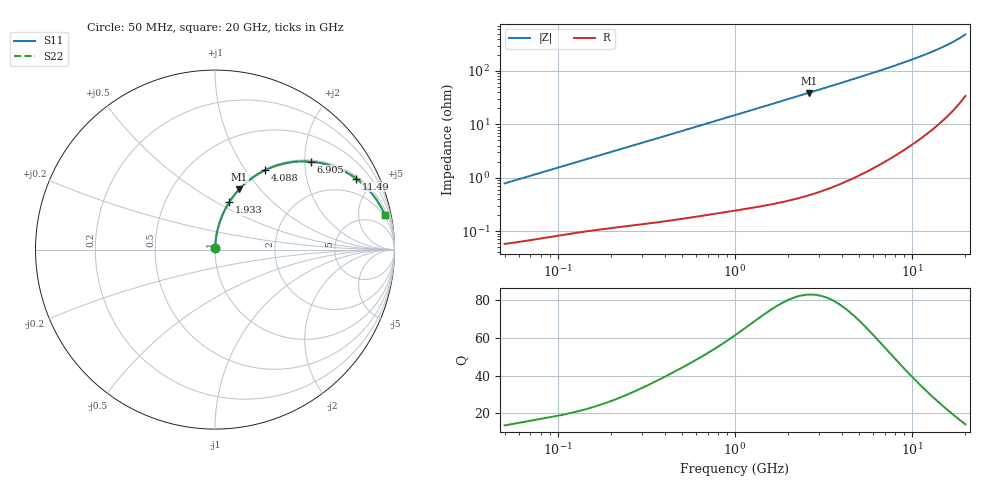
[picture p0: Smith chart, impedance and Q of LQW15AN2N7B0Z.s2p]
!Murata Part Number: LQW15AN2N7B0Z
!These Parameters are Measured in Series Mode Connection
!  o--[Z]--o
!Port1  Port2
!  o-------o
!Freq. Start=50[MHz] Stop=20[GHz], 401[Steps]
# Hz S RI R 50
!Freq.(Hz) S11(Real) S11(Imag) S21(Real) S21(Imag) S12(Real) S12(Imag) S22(Real) S22(Imag)
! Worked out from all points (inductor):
!   401 points, 50 MHz to 20 GHz, reference 50 ohm
!   read as one part in series: L = 2.48 nH near 51.52 MHz
!   highest Q = 83 at 2.608 GHz (marker M1), where L = 2.38 nH
!   S11 on the Smith chart (normalised r, x): 50 MHz: 1.00, +0.02; 1.933 GHz: 1.01, +0.58; 4.088 GHz: 1.02, +1.23; 6.905 GHz: 1.04, +2.15; 11.49 GHz: 1.12, +3.91; 20 GHz: 1.68, +9.64
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5e7  0.000638 0.00782  0.9994 -0.00782  0.9994 -0.00782  0.000638 0.00782
1.364002e8  0.0014 0.0208  0.9986 -0.0208  0.9986 -0.0208  0.0014 0.0208
2.33884e8  0.00246 0.0353  0.9975 -0.0353  0.9975 -0.0353  0.00246 0.0353
3.721004e8  0.00459 0.0556  0.9954 -0.0556  0.9954 -0.0556  0.00459 0.0556
6.285508e8  0.0106 0.0929  0.9894 -0.0929  0.9894 -0.0929  0.0106 0.0929
1e9  0.024 0.1453  0.976 -0.1453  0.976 -0.1453  0.024 0.1453
1.432596e9  0.0462 0.2031  0.9538 -0.2031  0.9538 -0.2031  0.0462 0.2031
1.932977e9  0.0795 0.2644  0.9205 -0.2644  0.9205 -0.2644  0.0795 0.2644
2.608132e9  0.1349 0.3356  0.8651 -0.3356  0.8651 -0.3356  0.1349 0.3356
2.728004e9  0.1457 0.3468  0.8543 -0.3468  0.8543 -0.3468  0.1457 0.3468
3.364474e9  0.2061 0.3984  0.7939 -0.3984  0.7939 -0.3984  0.2061 0.3984
4.087748e9  0.278 0.4415  0.722 -0.4415  0.722 -0.4415  0.278 0.4415
5.433528e9  0.4092 0.4842  0.5908 -0.4842  0.5908 -0.4842  0.4092 0.4842
6.905011e9  0.535 0.4899  0.465 -0.4899  0.465 -0.4899  0.535 0.4899
7.442007e9  0.575 0.4849  0.425 -0.4849  0.425 -0.4849  0.575 0.4849
9.178299e9  0.6833 0.4537  0.3167 -0.4537  0.3167 -0.4537  0.6833 0.4537
1.149051e10  0.7856 0.3959  0.2144 -0.3959  0.2144 -0.3959  0.7856 0.3959
1.334722e10  0.8425 0.3468  0.1575 -0.3468  0.1575 -0.3468  0.8425 0.3468
1.527346e10  0.8852 0.2979  0.1148 -0.2979  0.1148 -0.2979  0.8852 0.2979
1.721783e10  0.9163 0.2519  0.0837 -0.2519  0.0837 -0.2519  0.9163 0.2519
1.940974e10  0.9412 0.2045  0.0588 -0.2045  0.0588 -0.2045  0.9412 0.2045
2e10  0.9465 0.1925  0.0535 -0.1925  0.0535 -0.1925  0.9465 0.1925
